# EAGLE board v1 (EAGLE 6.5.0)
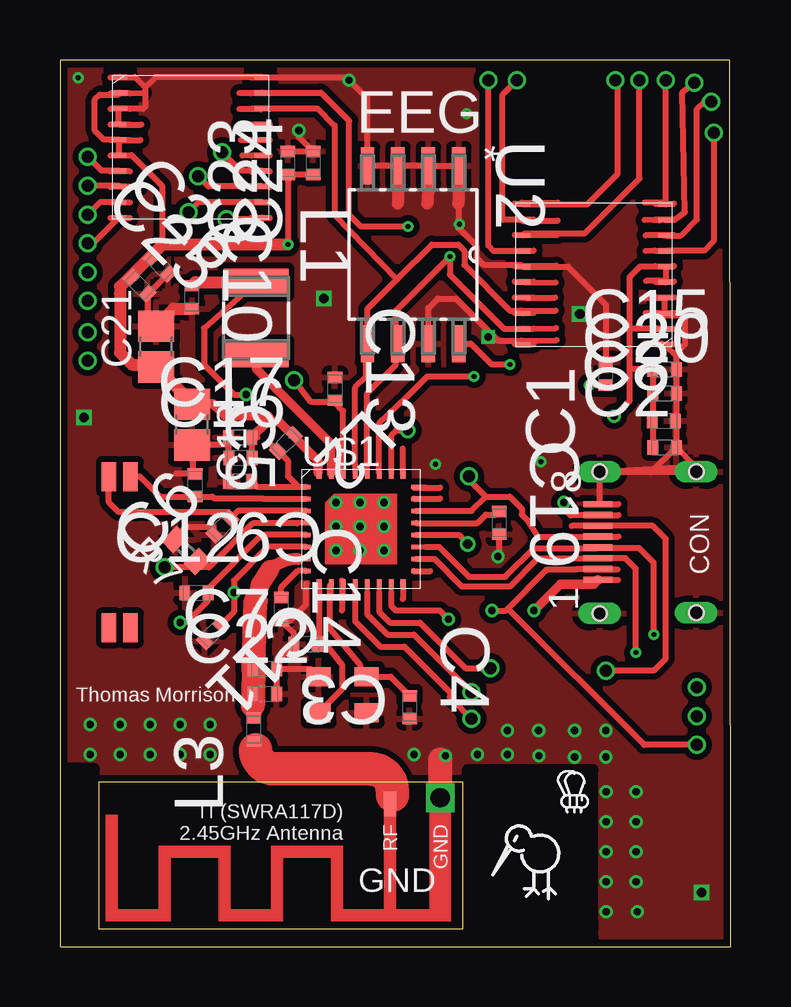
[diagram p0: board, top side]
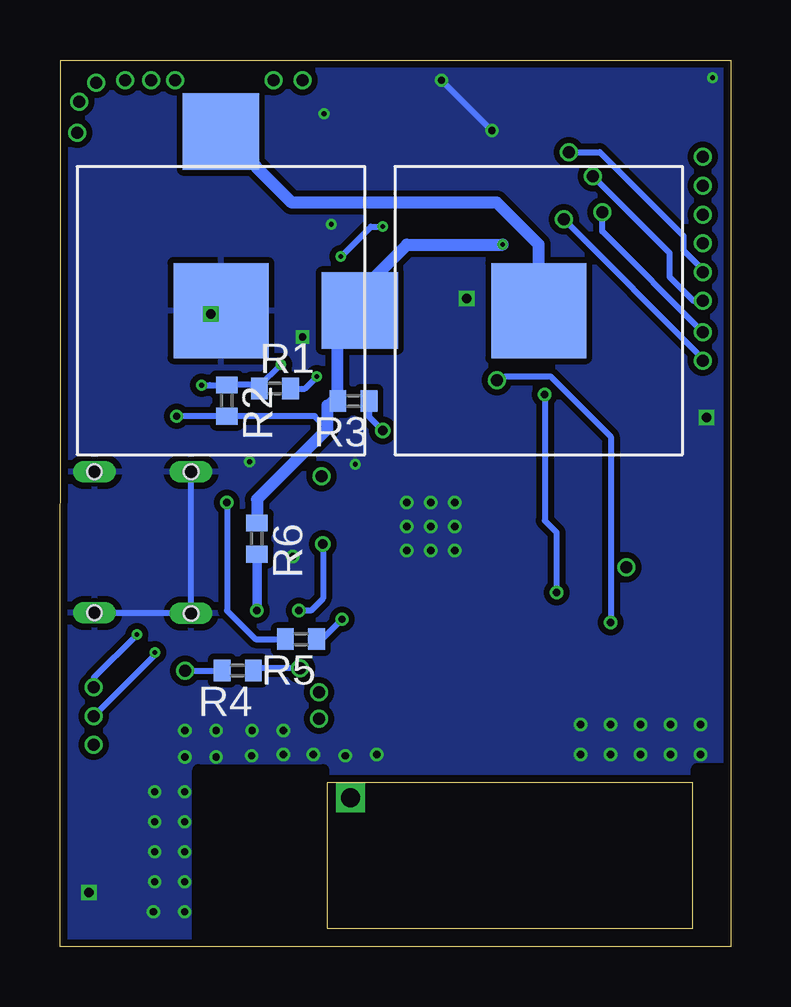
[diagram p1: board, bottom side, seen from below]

Size 27.97 x 36.94 mm. Coordinates in mm from the lower left corner, seen from the top.
Outline: 0.01,0 27.97,0 27.94,36.93 0,36.94 0.01,0
Copper layers (1*16): Top 0.035mm / dielectric 0.8mm / Bottom 0.035mm
Design rules "DRC *": minimum track width 0.15mm, minimum drill 0.2mm, track to track 0.15mm, track to pad 0.15mm, pad to pad 0.15mm, via to via 0.25mm, smd to smd 0.15mm, copper to edge 0.3mm, drill to drill 0.4mm, minimum pad ring 0mil, minimum via ring 0.125mm, stop-mask expansion 4mil, vias tented up to drill 0mil, thermal gap 10mil
tRestrict: area 17,0.8 to 22.2,7.3; area 0.4,0.5 to 1.4,7.4; area 17,0.4 to 22.2,1
bRestrict: area 17,0.8 to 22.2,7.3; area 0.4,0.5 to 1.4,7.4; area 17,0.4 to 22.2,1

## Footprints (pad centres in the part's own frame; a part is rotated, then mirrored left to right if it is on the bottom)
CAPC1005X60N = smd 0.457 x 0.61: 1 -0.483,0; 2 0.483,0
C0805 = smd 1.3 x 1.5: 1 -0.85,0; 2 0.85,0
SWRA117D_LEFT = drill 0.8 square: GND 0.45,0.25 | smd 0.508 x 1.016: RF 2.55,0.51
CAPC3225X127N = smd 1.118 x 2.692: 1 -1.499,0; 2 1.499,0
R0402 = smd 0.7 x 0.9: 1 -0.65,0; 2 0.65,0
SOIC127P798X216-8N = smd 1.549 x 0.559: 1 -3.708,1.905; 2 -3.708,0.635; 3 -3.708,-0.635; 4 -3.708,-1.905; 5 3.708,-1.905; 6 3.708,-0.635; 7 3.708,0.635; 8 3.708,1.905
CSR1010A05-IQQM-R = smd 0.186 x 0.4: AIO[0] -0.2,-0.9; AIO[1] -0.7,-0.9; AIO[2] -1.2,-0.9; I2C_SCL -0.2,3.7; I2C_SDA -0.7,3.7; PIO[0]/UART_TX 0.3,-0.9; PIO[1]/UART_RX 0.8,-0.9; PIO[2] 0.3,3.7; SMPS_LX -1.7,3.7; SPI_PIO# 0.8,3.7; VDD_CORE@1 -1.2,3.7; XTAL_16M_IN -1.7,-0.9 | smd 0.2 x 0.4: PIO[3]/SF_DIN 1.3,-0.9; PIO[11] 1.3,3.7; VDD_BAT_SMPS -2.2,3.7; XTAL_16M_OUT -2.2,-0.9 | smd 0.4 x 0.2: PIO[4]/SF_CS# 1.85,-0.35; PIO[10] 1.85,3.15; VDD_BAT -2.75,3.15; VDD_XTAL -2.75,-0.35 | smd 0.4 x 0.186: PIO[5]/DEBUG_CLK 1.85,0.15; PIO[6]/DEBUG_CS# 1.85,0.65; PIO[7]/DEBUG_MOSI 1.85,1.15; PIO[8]/DEBUG_MISO 1.85,2.15; PIO[9] 1.85,2.65; RF -2.75,0.15; VDD_CORE -2.75,1.15; VDD_PADS 1.85,1.65; VDD_REG_IN -2.75,0.65; WAKE -2.75,1.65; XTAL_32K_IN -2.75,2.15; XTAL_32K_OUT -2.75,2.65
8PIN_SMT_CONNECTOR = smd 0.26 x 1.2: 1 -1.32,2.83; 2 -0.87,2.83; 3 -0.42,2.83; 4 0.03,2.83; 5 0.48,2.83; 6 0.93,2.83; 7 1.38,2.83; 8 1.83,2.83 | drill 0.6 long: 9 3.18,2.755; 10 3.18,-1.27; 11 -2.695,-1.27; 12 -2.72,2.755 | hole 0.6: -2.72,2.755; -2.695,-1.27; 3.18,-1.27; 3.18,2.755
TSX3225 = smd 1 x 0.8: 1 -1,-0.75; 2 1,-0.75; 3 1,0.75; 4 -1,0.75
SSP-T7-F = smd 1.2 x 0.6: 1 -0.6,0.3; 2 5.7,0.3; 3 5.7,1.2; 4 -0.6,1.2
AD7997 = smd 0.6 x 0.2: P$01 -1.7,2.925; P$02 -1.7,2.275; P$03 -1.7,1.625; P$04 -1.75,0.975; P$05 -1.75,0.325; P$06 -1.75,-0.325; P$07 -1.75,-0.975; P$08 -1.75,-1.625; P$09 -1.75,-2.275; P$010 -1.75,-2.925; P$011 4.2,-2.925; P$012 4.2,-2.275; P$013 4.2,-1.625; P$014 4.2,-0.975; P$015 4.2,-0.325; P$016 4.2,0.325; P$017 4.2,0.975; P$018 4.2,1.625; P$019 4.2,2.275; P$020 4.2,2.925
BATTERY_2996 = smd 3.96 x 3.96: NEG 0,0 | smd 3.18 x 3.18: POS@2 7.463,0
TEST_POINT_0.5MM = drill 0.5: P$2 0,0

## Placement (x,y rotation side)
C1  1u  [CAPC1005X60N]  22.76,23.87 90 top
C2  1u  [CAPC1005X60N]  25.21,20.8 0 top
C3  15pF  [CAPC1005X60N]  10.24,12.6 180 top
C4  8.2pF  [CAPC1005X60N]  14.58,9.97 270 top
C5  10pF  [CAPC1005X60N]  5.64,19.23 270 top
C6  10pF  [CAPC1005X60N]  6.77,17.5 45 top
C7  0.5pF  [CAPC1005X60N]  8.55,11.57 0 top
C8  0.1u  [CAPC1005X60N]  25.18,21.9 0 top
C9  33p  [CAPC1005X60N]  7.51,19.38 180 top
C10  2u2  [CAPC1005X60N]  5.5,27.06 270 top
C11  470n  [CAPC1005X60N]  6.37,13.06 225 top
C12  470n  [CAPC1005X60N]  5.69,14.73 0 top
C13  150n  [CAPC1005X60N]  11.47,23.23 270 top
C14  470n  [CAPC1005X60N]  9.23,14.06 270 top
C15  1u  [CAPC1005X60N]  25.21,24.05 0 top
C16  47n  [CAPC1005X60N]  7.53,20.36 0 top
C17  2u2  [CAPC1005X60N]  7.52,21.21 0 top
C18  47u  [C0805]  5.51,21.75 270 top
C19  47n  [CAPC1005X60N]  18.31,17.66 270 top
C20  0.1u  [CAPC1005X60N]  25.21,23.05 0 top
C21  47u  [C0805]  4.01,25 90 top
C22  2.7 pF  [CAPC1005X60N]  8.54,10.53 0 top
C23  1u  [CAPC1005X60N]  9.51,32.65 90 top
C24  0.1u  [CAPC1005X60N]  10.56,32.65 90 top
C25  1u  [CAPC1005X60N]  3.31,27.54 315 top
C26  0.1u  [CAPC1005X60N]  4.17,28.37 315 top
GND  ANTENNA_1LEFT  [SWRA117D_LEFT]  16.31,6.45 180 top
L1  4.7uH  [CAPC3225X127N]  8.18,26.19 270 top
L2  Ferrite Core (MMZ1005Y152C)  [CAPC1005X60N]  9.42,20.98 225 top
L3  Ferrite Core (MMZ1005Y152C)  [CAPC1005X60N]  8.09,9.04 90 top
R1  10K  [R0402]  19.01,23.25 0 bottom
R2  10K  [R0402]  21.01,22.75 270 bottom
R3  10K  [R0402]  15.74,22.73 180 bottom
R4  10K  [R0402]  20.56,11.5 180 bottom
R5  10K  [R0402]  17.92,12.81 180 bottom
R6  10K  [R0402]  19.76,17 270 bottom
R7  10K  [R0402]  5.26,16.5 135 top
U2  AT24C512C-SHD-B  [SOIC127P798X216-8N]  14.73,28.83 270 top
U$1  CSR1010A05-IQQM-R  [CSR1010A05-IQQM-R]  13.01,16 0 top
U$2  8PIN_SMT_CONNECTOR  [8PIN_SMT_CONNECTOR]  25.26,16.6 90 top
U$3  TSX3225  [TSX3225]  11.79,10.49 0 top
U$4  SSP-T7-F  [SSP-T7-F]  1.74,18.98 270 top
U$5  AD7997  [AD7997]  23.51,28 180 top
U$6  AD7997  [AD7997]  4.21,33.3 0 top
U$7  BATTERY_2996  [BATTERY_2996]  21.26,26.5 90 bottom
U$8  BATTERY_2996  [BATTERY_2996]  8.01,26.5 180 bottom
U$9  TEST_POINT_0.5MM  [TEST_POINT_0.5MM]  1.16,28.1 0 top
U$10  TEST_POINT_0.5MM  [TEST_POINT_0.5MM]  1.16,26.9 0 top
U$11  TEST_POINT_0.5MM  [TEST_POINT_0.5MM]  1.16,25.6 0 top
U$12  TEST_POINT_0.5MM  [TEST_POINT_0.5MM]  1.16,24.4 0 top
U$13  TEST_POINT_0.5MM  [TEST_POINT_0.5MM]  1.16,32.9 0 top
U$14  TEST_POINT_0.5MM  [TEST_POINT_0.5MM]  1.16,31.7 0 top
U$15  TEST_POINT_0.5MM  [TEST_POINT_0.5MM]  1.16,30.5 0 top
U$16  TEST_POINT_0.5MM  [TEST_POINT_0.5MM]  1.16,29.3 0 top
U$17  TEST_POINT_0.5MM  [TEST_POINT_0.5MM]  17.86,36.1 0 top
U$18  TEST_POINT_0.5MM  [TEST_POINT_0.5MM]  24.16,36.1 0 top
U$19  TEST_POINT_0.5MM  [TEST_POINT_0.5MM]  19.06,36.1 0 top
U$20  TEST_POINT_0.5MM  [TEST_POINT_0.5MM]  23.16,36.1 0 top
U$21  TEST_POINT_0.5MM  [TEST_POINT_0.5MM]  27.26,33.9 0 top
U$22  TEST_POINT_0.5MM  [TEST_POINT_0.5MM]  27.16,35.2 0 top
U$23  TEST_POINT_0.5MM  [TEST_POINT_0.5MM]  26.46,36 0 top
U$24  TEST_POINT_0.5MM  [TEST_POINT_0.5MM]  25.26,36.1 0 top
U$25  TEST_POINT_0.5MM  [TEST_POINT_0.5MM]  17.06,19.6 0 top
U$26  TEST_POINT_0.5MM  [TEST_POINT_0.5MM]  26.56,8.4 0 top
U$27  TEST_POINT_0.5MM  [TEST_POINT_0.5MM]  26.56,10.8 0 top
U$28  TEST_POINT_0.5MM  [TEST_POINT_0.5MM]  26.56,9.6 0 top
U$29  TEST_POINT_0.5MM  [TEST_POINT_0.5MM]  17.16,9.5 0 top
U$30  TEST_POINT_0.5MM  [TEST_POINT_0.5MM]  17.16,10.6 0 top
U$31  TEST_POINT_0.5MM  [TEST_POINT_0.5MM]  4.36,15.8 0 top

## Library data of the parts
C1 C2 C5 C6 C8-C15 C19 C20 C23-C26 L2 L3 = AVX_By_element14_Batch_1; MPN: UQCL2A100JAT2A/500; OC_FARNELL: -; OC_NEWARK: 32T8791; SUPPLIER: AVX; TOLERANCE: ±5%; VOLTAGERATING: 200V
C3 = AVX_By_element14_Batch_1; MPN: UQCL2A150JAT2A/500; OC_FARNELL: -; OC_NEWARK: 32T8795; SUPPLIER: AVX; TOLERANCE: ±5%; VOLTAGERATING: 200V
C4 = AVX_By_element14_Batch_1; MPN: UQCL2A8R2CAT2A/500; OC_FARNELL: -; OC_NEWARK: 32T8828; SUPPLIER: AVX; TOLERANCE: ±.25 pF; VOLTAGERATING: 200V
C7 C22 = AVX_By_element14_Batch_1; MPN: UQCL2A0R5BAT2A/500; OC_FARNELL: -; OC_NEWARK: 32T8767; SUPPLIER: AVX; TOLERANCE: ±.1 pF; VOLTAGERATING: 200V
C16 C17 = AVX_By_element14_Batch_1; MPN: UQCL2A1R0BAT2A/500; OC_FARNELL: -; OC_NEWARK: 32T8778; SUPPLIER: AVX; TOLERANCE: ±.1 pF; VOLTAGERATING: 200V
C18 C21 = resistor
GND = ant-planar-1
L1 = AVX_By_element14_Batch_1; MPN: 12107C102JAT2A; OC_FARNELL: -; OC_NEWARK: 56J0850; SUPPLIER: AVX; TOLERANCE: ±5%; VOLTAGERATING: 500V
R1-R7 = rcl
U2 = ATMEL-AT24C512C-SHD-B; MPN: AT24C512C-SHD-B; OC_FARNELL: 1972003; OC_NEWARK: 68T4124; PACKAGE: 8SOIC-Wide; SUPPLIER: ATMEL
U$1 = CSR1010A05
U$2 = MINI_SMT_8_PIN_CONNECTOR
U$3 = TSX3225
U$4 = SSP-T7-F
U$5 U$6 = AD7997
U$7 U$8 = BATTERY_2996_2
U$9-U$31 = TEST_POINT_0.5mm

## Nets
GND: C1.2 C2.2 C3.2 C4.2 C6.1 C7.2 C8.2 C9.2 C10.2 C11.2 C12.1 C13.1 C14.2 C15.2 C16.1 C17.1 C18.2 C19.2 C20.2 C21.2 C22.2 C23.2 C24.2 C25.2 C26.2 R7.2 U2.1 U2.2 U2.3 U2.4 U2.7 U$2.8 U$2.9 U$2.10 U$2.11 U$2.12 U$3.2 U$3.4 U$5.P$01 U$5.P$03 U$5.P$04 U$5.P$015 U$5.P$020 U$6.P$01 U$6.P$03 U$6.P$04 U$6.P$020 U$7.NEG
N$1: U$1.PIO[11]
N$2: U$1.PIO[9]
N$3: R1.2 U$1.PIO[2]
N$4: C1.1 R1.1 R2.1 U2.8
N$5: U$1.PIO[10]
N$12: U$6.P$08 U$14.P$2
N$14: U$6.P$07 U$13.P$2
N$16: U$6.P$09 U$15.P$2
N$18: U$1.PIO[8]/DEBUG_MISO U$2.5 U$25.P$2
N$19: L1.2 U$1.SMPS_LX
N$20: R4.2 U$2.6
N$23: U$1.PIO[3]/SF_DIN
N$25: U$1.PIO[4]/SF_CS#
N$26: C5.2 U$1.XTAL_32K_OUT U$4.4
N$27: C6.2 U$1.XTAL_32K_IN U$4.1
N$28: U$1.AIO[1] U$29.P$2
N$29: C3.1 U$1.XTAL_16M_OUT U$3.1
N$30: C4.1 U$1.XTAL_16M_IN U$3.3
N$31: U$1.PIO[6]/DEBUG_CS# U$2.4 U$27.P$2
N$32: C9.1 L2.2 U$1.VDD_BAT
N$33: U$1.AIO[0] U$30.P$2
N$34: L3.1
N$35: C14.1 U$1.VDD_XTAL
N$36: R5.2 U$2.7
N$37: R4.1 U$1.PIO[0]/UART_TX
N$38: R5.1 U$1.PIO[1]/UART_RX
N$39: C10.1 C11.1 L1.1 U$1.VDD_REG_IN
N$40: R6.2 U$2.1
N$43: C7.1 C22.1 L3.2 U$1.RF
N$45: R3.1 U$1.SPI_PIO#
N$46: U$5.P$014 U$17.P$2
N$49: R7.1 U$1.WAKE U$31.P$2
N$50: U$1.PIO[7]/DEBUG_MOSI U$2.2 U$26.P$2
N$51: U$1.PIO[5]/DEBUG_CLK U$2.3 U$28.P$2
N$73: U$5.P$012 U$19.P$2
N$82: U$5.P$013 U$18.P$2
N$83: U$5.P$011 U$20.P$2
N$87: C19.1 U$1.VDD_PADS
N$90: U$6.P$010 U$16.P$2
N$106: U$6.P$011 U$12.P$2
N$117: U$6.P$012 U$11.P$2
N$118: U$6.P$013 U$10.P$2
N$137: U$6.P$014 U$9.P$2
N$138: U$7.POS@2 U$8.NEG
N$139: U$5.P$07 U$21.P$2
N$140: U$5.P$08 U$22.P$2
N$141: U$5.P$09 U$23.P$2
N$142: U$5.P$010 U$24.P$2
N$151: U$5.P$017
N$152: U$5.P$016
SCL: U2.6 U$1.I2C_SCL U$5.P$019 U$6.P$019
SDA: U2.5 U$1.I2C_SDA U$5.P$018 U$6.P$018
VDD: C2.1 C8.1 C15.1 C16.2 C17.2 C18.1 C20.1 C21.1 C23.1 C24.1 C25.1 L2.1 R2.2 R3.2 R6.1 U$1.VDD_BAT_SMPS U$5.P$02 U$5.P$05 U$5.P$06 U$6.P$02 U$6.P$05 U$6.P$06 U$8.POS@2
VDD_CORE: C12.2 C13.2 U$1.VDD_CORE U$1.VDD_CORE@1

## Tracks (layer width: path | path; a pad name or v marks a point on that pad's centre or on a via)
GND  (via drill 0.2, 0.3, 0.4)
  Top 0.1: v11.51,16.5 11.51,16.25 11.26,16
  Top 0.125: 11.26,16 11.16,16
  Top 0.25: C6.1 6.39,17.5 5.26,17.5 4.8,17.04 R7.2 | U2.7 15.36,26.61 15.76,27 16.51,27 18.26,25.25 19.23,25.25 19.31,25.18 U$5.P$020 | C7.2 9.03,11.87 C3.2 9.75,13.05 C14.2 9.59,13.58 10.26,14.25 10.26,15.1 10.28,15.12 | C7.2 10.46,11.57 U$3.4 | 24.39,27.01 25.26,27 U$5.P$04 25.21,26.98 U$5.P$03 25.28,26.3 26.06,26.3 26.06,25.1 25.69,24.73 25.69,24.59 | C7.2 9.02,11.56 C22.2 | 7.01,20.9 5.56,20.9 | 5.56,20.9 C18.2 | 7.01,20.9 7.01,19.9 C9.2 C16.1 | C17.1 7.03,20.92 7.01,20.9 | C1.2 22.76,26.75 21.18,28.32 U$5.P$015 19.23,28.4 17.66,28.4 17.36,28.7 17.36,29.2 16.61,29.95 16.61,30.96 | U2.1 U2.2 U2.3 U2.4 12.82,35.44 12.72,35.44 v12.06,36.1 11.93,36.23 U$6.P$020 3.98,36.23 3.56,35.8 | C19.2 18.31,16.3 v18.26,16.25 | C2.2 C15.2 25.69,24.59 | 26.64,19.84 26.47,20.02 | 26.47,20.02 C2.2 | 24.64,19.75 C2.2 | C26.2 3.79,27.3 3.66,27.3 3.65,27.29 C25.2 3.65,26.21 C21.2 | C23.2 C24.2 9.96,33.73 v9.96,34 | U$6.P$04 2.46,34.88 U$6.P$03 2.53,34.9 3.46,34.9 3.56,35 3.56,35.8 | U$6.P$01 3.13,36.23 3.56,35.8 | U$5.P$01 25.69,24.59 | U$2.9 U$2.10 | U$2.8 22.5,18.5 U$2.9 | v16.66,30.1 16.66,30 | U$2.9 26.47,20.02 | 5.56,20.9 5.56,19.7 4.86,19.7
  Top 0.5: U2.3 14.09,30.97 | U2.2 15.32,30.96 | U2.1 16.61,30.96 | C21.2 4.73,26.58 C10.2
  Top 1: 15.86,6 15.86,7.8
  Bottom 0.25: v9.96,34 v12.06,36.1 | U$2.11 22.53,13.9 | 22.53,13.9 U$2.12 | 22.53,13.9 22.5,13.93 U$2.9
  other vias: 16.07,7.96 6.26,8 5.01,8 3.76,8 2.51,8 1.26,8 14.76,8 1.26,9.25 2.51,9.25 3.76,9.25 5.01,9.25 6.26,9.25 24.02,6.46 24.02,5.21 24.02,3.96 24.02,2.71 22.77,1.46 22.77,2.71 22.77,3.96 22.77,5.21 22.77,6.46 1.01,22.05 11.01,27 26.76,2.25 21.68,26.35 13.51,18.5 13.51,17.5 13.51,16.5 12.51,17.5 12.51,18.5 12.51,16.5 11.51,17.5 11.51,18.5 24.07,1.46 17.86,25.4 22.76,7.9 22.76,9 21.46,9 21.46,7.9 19.96,9 19.97,7.96 17.41,8 18.66,8 18.66,9 16.96,34.7 15.66,20.1 20.06,20.2 0.76,36.2
  pour Bottom (isolate 0.25): 0.16,0.2 27.76,0.2 27.86,36.85 0.16,36.75
  pour Top (isolate 0.25): 0.26,0.2 27.76,0.2 27.86,36.7 27.86,36.8 0.16,36.8
N$3  (via drill 0.2)
  Top 0.25: U$1.PIO[2] 13.31,21.8 14.46,22.89 15.31,23.75 v17.26,23.75
  Bottom 0.25: R1.2 17.76,23.25 v17.26,23.75
N$4  (via drill 0.2)
  Top 0.25: C1.1 v22.06,23.39 | U2.8 17.13,25.12 18.01,24.25 v18.76,24.25
  Bottom 0.25: v22.06,23.39 arc-1 R2.1 20.01,23.4 R1.1 19.66,23.35 v18.76,24.25
N$12
  Top 0.25: U$6.P$08 2.43,31.7 U$14.P$2
N$14
  Top 0.25: U$6.P$07 1.73,32.33 U$13.P$2
N$16
  Top 0.25: U$15.P$2 1.68,31.02 U$6.P$09
N$17
  Top 0.25: 14.3,19.7 14.3,20.31
N$18
  Top 0.25: U$1.PIO[8]/DEBUG_MISO 17.16,18.15 17.76,18.75 | 17.76,18.75 18.76,18.75 19.26,18.25 19.26,18 19.51,17.75 19.95,17.07 19.97,17.08 U$2.5 | U$25.P$2 17.06,19.45 17.76,18.75
N$19
  Top 0.3: 8.18,24.33 L1.2
  Top 0.35: U$1.SMPS_LX 11.31,20.95 8.18,24.08 L1.2
N$20  (via drill 0.5)
  Top 0.25: v22.76,11.5 24.76,11.5 25.26,12 25.26,17 24.73,17.53 U$2.6 21.34,17.53
  Bottom 0.25: v22.76,11.5 R4.2
N$21
  Top 0.25: 14.3,15.15 14.3,14.47
N$24
  Top 0.25: 14.75,15.64 15.44,15.64
N$26
  Top 0.25: U$1.XTAL_32K_OUT 8.48,18.65 8.46,18.67 6.44,18.67 6.36,18.74 C5.2 4.18,18.74 3.34,19.58 U$4.4
N$27
  Top 0.25: U$1.XTAL_32K_IN 7.42,18.15 C6.2 7.01,18.09 3.16,18.09 3.16,18.1 2.46,18.1 2.04,18.52 U$4.1
N$28
  Top 0.25: 12.31,14.75 12.31,13.55 13.36,12.5 14.36,12.5 16.26,10.6 16.26,10.4 U$29.P$2
N$29
  Top 0.25: U$1.XTAL_16M_OUT 10.81,12.95 10.88,12.85 | 10.88,12.85 11.76,11.75 11.76,10.71 U$3.1 | C3.1 10.72,12.69 10.88,12.85
N$30
  Top 0.25: U$1.XTAL_16M_IN 11.26,15.05 11.26,13.25 12.51,11.75 12.51,11.52 U$3.3 12.77,11.24 12.76,11.25 13.78,11.25 C4.1
N$31  (via drill 0.2)
  Top 0.25: v24.76,13 24.76,16 24.15,16.61 22.45,16.61 U$2.4 22.4,16.6 19.76,16.6 18.56,15.4 17.06,15.4 15.81,16.65 15.26,16.65
  Bottom 0.25: v24.76,13 26.56,11.2 U$27.P$2
N$32
  Top 0.25: 8.84,20.88 L2.2 9.26,20.5 9.51,20.25 9.51,19.6 9.96,19.15 U$1.VDD_BAT 8.22,19.15 C9.1
N$33
  Top 0.25: 12.81,14.75 12.81,13.85 13.66,13 14.76,13 U$30.P$2
N$35
  Top 0.25: U$1.VDD_XTAL 9.91,15.65 9.23,14.97 C14.1
N$36  (via drill 0.3)
  Top 0.25: v21.01,18.5 21.01,18.25 21.3,17.95 21.33,17.98 U$2.7
  Bottom 0.25: v21.01,18.5 21.01,14 19.81,12.81 R5.2
N$37  (via drill 0.5)
  Top 0.25: 13.31,14.75 13.31,13.95 13.76,13.5 15.01,13.5 16.91,11.6 v17.96,11.6
  Bottom 0.25: v17.96,11.6 19.81,11.6 arc-90 R4.1
N$38  (via drill 0.3)
  Top 0.25: 13.81,14.75 13.81,14.2 14.01,14 15.84,14 v16.2,13.63
  Bottom 0.25: R5.1 17.03,12.81 v16.2,13.63
N$39  (via drill 0.3)
  Top 0.25: U$1.VDD_REG_IN 8.66,16.65 7.26,15.25 v7.26,14.75 7.26,13.95 C11.1 | L1.1 6.01,25.77 6.01,24.25 7.26,23 v7.76,23
  Top 0.5: C10.1 5.65,27.69 L1.1
  Bottom 0.25: v7.76,23 7.76,17.75 7.26,17.25 v7.26,14.75
N$40  (via drill 0.3)
  Top 0.4: U$2.1 22.26,15.1 20.86,15.1 v19.76,14
  Bottom 0.4: R6.2 v19.76,14
N$43
  Top 0.25: 8.05,10.04 L3.2
  Top 0.5: 9.91,16.15 arc90 8.16,14.4
  Top 1: 8.16,14.4 C7.1 C22.1 8.05,10.04
N$45  (via drill 0.4)
  Top 0.25: v14.51,21.5 14.01,21.5 13.81,21.3 U$1.SPI_PIO#
  Bottom 0.25: R3.1 15.09,22.08 v14.51,21.5
N$46
  Top 0.25: U$5.P$014 18.08,28.98 17.86,29.2 U$17.P$2
N$49
  Top 0.25: 9.91,17.65 9.89,17.63 8.04,17.63 6.26,15.85 | 6.26,15.85 R7.1 | 6.26,15.85 6.21,15.8 U$31.P$2
N$50  (via drill 0.3, 0.4)
  Top 0.25: v18.01,14 18.6,14 18.68,14.08 | U$1.PIO[7]/DEBUG_MOSI 16.63,17.15 v17.01,16.77 | 18.68,14.08 20.25,15.65 20.31,15.71 21.53,15.71 21.55,15.73 U$2.2 | U$26.P$2 24.36,8.4 18.68,14.08
  Bottom 0.25: v17.01,16.77 17.01,14.5 17.51,14 v18.01,14
N$51  (via drill 0.2)
  Top 0.25: U$1.PIO[5]/DEBUG_CLK 15.61,16.15 16.76,15 18.76,15 19.94,16.18 U$2.3 23.58,16.18 24.01,15.75 v24.01,12.25
  Bottom 0.25: U$28.P$2 24.01,12.15 v24.01,12.25
N$73
  Top 0.25: U$5.P$012 18.48,30.27 18.46,30.3 18.46,35.5 U$19.P$2
N$82
  Top 0.25: U$5.P$013 19.38,29.7 21.86,29.7 24.16,32 U$18.P$2
N$83
  Top 0.25: U$5.P$011 21.98,30.93 23.26,32.2 23.26,35.8 U$20.P$2
N$86
  Top 0.25: 11.76,15.25 11.76,14
N$87
  Top 0.25: U$1.VDD_PADS 17.4,17.64 17.76,18 18.17,18 C19.1
N$88
  Top 0.25: 14.74,19.12 15.86,19.12
N$89
  Top 0.25: 14.75,18.66 15.86,18.66
N$90
  Top 0.25: U$16.P$2 1.38,29.3 U$6.P$010
N$91
  Top 0.25: 19.26,25.25 20.71,25.27
N$92
  Top 0.25: 19.26,26.5 20.67,26.5
N$93
  Top 0.25: 19.26,30.25 20.76,30.25
N$94
  Top 0.25: 19.42,29.66 20.73,29.64
N$95
  Top 0.25: 20.7,28.37 19.37,28.35
N$96
  Top 0.25: 19.42,27.66 20.66,27.68
N$97
  Top 0.25: 19.44,27.04 20.64,27.04
N$98
  Top 0.25: 25.12,25.11 24.36,25.11
N$99
  Top 0.25: 25.19,26.39 24.42,26.39
N$100
  Top 0.25: 25.26,27.75 24.43,27.74
N$101
  Top 0.25: 24.76,29 24.42,28.98
N$102
  Top 0.25: 25.15,29.63 24.41,29.63
N$103
  Top 0.25: 25.01,30.25 24.38,30.27
N$104
  Top 0.25: 25.26,31 24.38,31
N$105
  Top 0.25: 19.26,31 20.76,31
N$106  (via drill 0.5)
  Top 0.25: U$6.P$011 8.41,30.3 v6.96,30.3
  Bottom 0.25: v6.96,30.3 1.16,24.5 U$12.P$2
N$110
  Top 0.25: 2.52,35.55 3.46,35.56
N$113
  Top 0.25: 2.47,34.24 3.39,34.24
N$117  (via drill 0.5)
  Top 0.25: v5.36,30.6 5.78,31.02 U$6.P$012
  Bottom 0.25: U$11.P$2 5.36,29.8 v5.36,30.6
N$118  (via drill 0.5)
  Top 0.25: U$6.P$013 6.18,31.68 v5.76,32.1
  Bottom 0.25: v5.76,32.1 2.56,28.9 2.56,27.9 1.56,26.9 U$10.P$2
N$119
  Top 0.25: 22.49,18.43 23.3,18.43
N$120
  Top 0.25: 22.49,17.98 23.3,17.98
N$121
  Top 0.25: 22.49,17.07 23.29,17.07
N$122
  Top 0.25: 22.47,15.72 23.25,15.72
N$123
  Top 0.25: 22.47,15.28 23.28,15.28
N$124
  Top 0.25: 14.29,20.09 14.3,20.1 14.3,20.76
N$125
  Top 1.4: 13.86,6.3 13.86,6.5 arc90 12.96,7.4 8.96,7.4 arc-90 8.16,8.2
N$126
  Top 0.8: 8.16,14.3 8.36,15.1 8.76,15.7
N$127
  Top 0.25: 8.41,34.25 7.49,34.25
N$128
  Top 0.25: 8.38,34.88 7.48,34.89
N$129
  Top 0.25: 8.34,35.55 7.48,35.55
N$135
  Top 0.25: 8.34,33.6 7.55,33.6
N$136
  Top 0.25: 2.58,31.65 3.32,31.65
N$137  (via drill 0.5)
  Top 0.25: U$6.P$014 7.53,32.33 v6.76,33.1
  Bottom 0.25: v6.76,33.1 5.46,33.1 1.96,29.6 1.96,29 1.16,28.2 U$9.P$2
N$138
  Bottom 0.5: U$8.NEG 8.01,29.25 9.76,31 18.29,31 U$7.POS@2
N$139
  Top 0.25: U$5.P$07 25.28,29 26.86,29 27.26,29.4 U$21.P$2
N$140
  Top 0.25: U$5.P$08 25.88,29.62 26.56,30.3 26.56,34.9 26.86,35.2 U$22.P$2
N$141
  Top 0.25: U$5.P$09 25.63,30.27 26.06,30.6 25.96,35.6 U$23.P$2
N$142
  Top 0.25: U$5.P$010 U$24.P$2
N$143
  Top 0.25: 8.44,32.95 7.61,32.97
SCL  (via drill 0.2)
  Top 0.25: 12.81,20.05 12.81,23.05 14.01,24.25 14.01,25.29 U2.6 14.09,25.41 14.01,25.5 14.01,26.5 v16.26,28.75 16.26,28 18.51,25.75 19.28,25.75 | 19.28,25.75 U$5.P$019 | 19.28,25.75 20.69,25.77 | v14.51,30 12.56,30 12.06,30.5 12.06,34.4 10.88,35.58 U$6.P$019
  Bottom 0.25: v16.26,28.75 15.01,30 v14.51,30
SDA
  Top 0.25: 12.31,20.05 12.31,23.3 12.76,23.75 12.76,25.06 U2.5 12.82,26.57 14.06,27.8 | 14.06,27.8 15.51,29.25 16.61,29.25 16.86,29 16.86,28.4 18.76,26.5 19.18,26.5 U$5.P$018 | 14.06,27.8 11.46,30.5 11.46,34.2 10.73,34.92 U$6.P$018
VDD  (via drill 0.2, 0.3)
  Top 0.25: 8.88,21.88 8.76,22 | U$5.P$02 25.18,25.75 23.76,25.75 | 23.76,25.75 23.76,27.9 24.18,28.32 U$5.P$06 U$5.P$05 | C16.2 8.01,21.2 C17.2 8.22,21.21 | v23.11,22.1 23.76,22.75 23.76,24.1 | 23.76,24.1 23.76,25.75 | 23.76,24.1 23.81,24.05 C15.1 C20.1 C2.1 24.72,21.88 C8.1 | 4.26,29.25 4.26,31.7 2.98,32.98 U$6.P$06 2.46,33.6 | 2.46,33.6 U$6.P$05 1.83,33.62 1.46,34 1.46,35.3 1.66,35.5 2.43,35.5 U$6.P$02 | v9.51,29.25 C23.1 C24.1 | C21.1 4.01,24.25 | C25.1 2.51,27.42 2.51,27.2 | 2.46,33.6 3.36,33.6 | U$1.VDD_BAT_SMPS 10.81,19.75 10.76,19.75
  Top 0.4: 6.13,22.62 6.37,22.62 6.88,22.11 8.65,22.11 8.76,22 | 9.68,21.32 10.76,20.25 10.76,19.75 | C17.2 8.66,21.88 8.88,21.88 9.13,21.88 9.68,21.32 | L2.1 9.68,21.32
  Top 0.5: 6.13,22.62 5.53,22.62 C18.1 5.51,22.65 C21.1 | 4.01,24.25 3.01,24.25 2.51,24.75 2.51,27.2 2.51,27.5 4.26,29.25 v9.51,29.25
  Bottom 0.25: 16.57,22.55 16.76,22.55 16.82,22.55 | v23.11,22.1 R2.2 17.35,22.1 16.82,21.57
  Bottom 0.5: 16.82,22.55 16.82,21.57 19.76,18.63 R6.1 | 16.76,22.55 16.58,22.73 R3.2 16.39,25.58 U$8.POS@2 15.51,26.54 15.51,27.25 13.51,29.25 v9.51,29.25
VDD_CORE  (via drill 0.3, 0.5)
  Top 0.25: 11.81,20.05 11.81,22.31 11.42,22.7 | v5.01,13.5 5.26,13.5 6.17,14.42 C12.2 6.17,14.92 8.41,17.15 U$1.VDD_CORE | v9.76,23.6 10.46,22.7 11.42,22.7 | 11.42,22.7 C13.2
  Bottom 0.25: v5.01,13.5 5.01,21.25 7.51,23.75 9.41,23.75 v9.76,23.6

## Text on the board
tPlace: EEG | CON | Thomas Morrison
